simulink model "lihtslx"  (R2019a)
settings: configuration reference "configurationSettings" (kept in a data dictionary, not in this file)
libraries: liulib x1

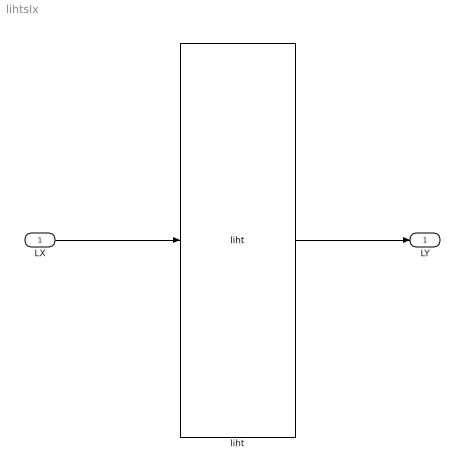
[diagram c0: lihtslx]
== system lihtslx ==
  LX : Inport  OutDataTypeStr=Bus: LXbus  PortDimensions=1  SampleTime=0
  liht : liulib/liht  SystemSampleTime=-1
  LY : Outport  OutDataTypeStr=Bus: LYbus  PortDimensions=1  SampleTime=0
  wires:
  LX/1 -> liht/1
  liht/1 -> LY/1
